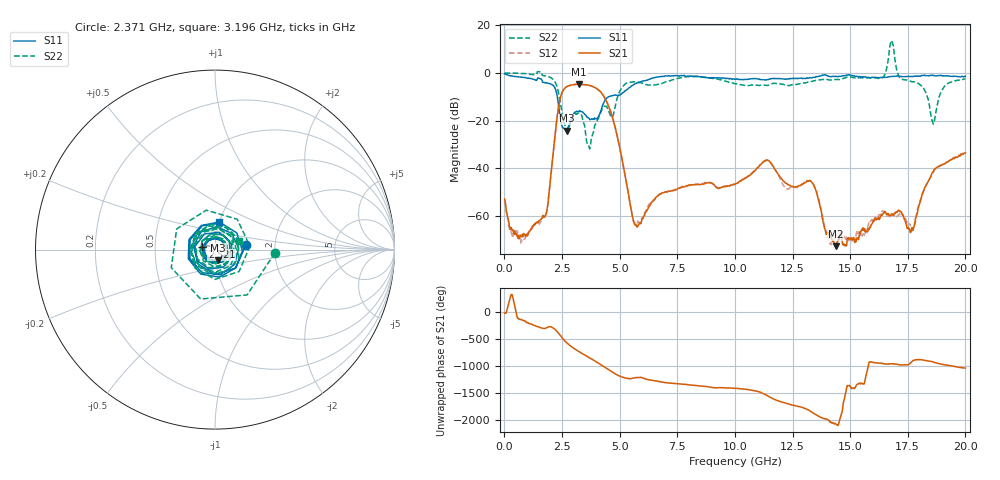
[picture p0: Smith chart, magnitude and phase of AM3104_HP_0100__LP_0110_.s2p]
!Created with skrf (http://scikit-rf.org).
# Hz S RI R 50.0
!freq ReS11 ImS11 ReS21 ImS21 ReS12 ImS12 ReS22 ImS22
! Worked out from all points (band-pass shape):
!   1601 points, 10 MHz to 20 GHz, reference 50 ohm
!   highest |S21| = -4.74 dB at 3.246 GHz (marker M1); lowest = -72.7 dB at 14.37 GHz (marker M2)
!   |S21| within 3 dB of the highest: 2.525 GHz to 4.153 GHz (1.628 GHz wide, 48.8 % of centre)
!   lowest |S11| = -24.3 dB at 2.696 GHz (marker M3), VSWR 1.13, Z = 51.4 - j6.05 ohm
!   |S11| at or under -10 dB: 2.297 GHz to 4.518 GHz (2.221 GHz wide, 65.2 % of centre)
!   |S22| runs from -31.9 to 13.6 dB; largest |S21 - S12| = 0.032
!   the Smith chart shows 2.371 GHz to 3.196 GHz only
!   S11 on the Smith chart (normalised r, x): 2.371 GHz: 1.41, +0.07; 2.521 GHz: 0.87, +0.02; 3.196 GHz: 1.00, +0.32
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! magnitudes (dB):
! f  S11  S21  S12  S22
! 10 MHz  -0.4  -52.9  -54.0  0.0
! 784.6 MHz  -1.8  -68.2  -70.4  -0.2
! 1.759 GHz  -4.1  -60.1  -60.5  -1.2
! 2.371 GHz  -15.2  -13.2  -13.2  -9.5
! 2.521 GHz  -22.9  -7.8  -7.9  -17.7
! 2.696 GHz  -24.3  -5.8  -5.8  -23.0
! 3.196 GHz  -16.2  -4.8  -4.9  -16.9
! 3.246 GHz  -16.3  -4.7  -4.8  -17.1
! 3.346 GHz  -16.3  -4.8  -4.9  -17.7
! 3.658 GHz  -19.0  -5.2  -5.3  -30.5
! 4.545 GHz  -9.9  -14.6  -14.6  -16.6
! 5.682 GHz  -4.5  -63.9  -63.7  -3.7
! 6.682 GHz  -1.6  -51.3  -51.4  -4.8
! 10.01 GHz  -2.7  -46.8  -46.7  -4.5
! 11.38 GHz  -2.9  -36.6  -36.8  -5.2
! 13.34 GHz  -2.1  -46.0  -46.0  -3.6
! 14.37 GHz  -1.4  -72.7  -68.7  -2.8
! 16.36 GHz  -1.9  -59.5  -58.5  -2.2
! 16.68 GHz  -1.6  -59.4  -60.3  7.2
! 17.69 GHz  -1.6  -65.1  -66.0  -3.7
! 18.6 GHz  -1.1  -41.5  -41.9  -21.3
! 20 GHz  -1.5  -33.6  -33.1  -2.5
